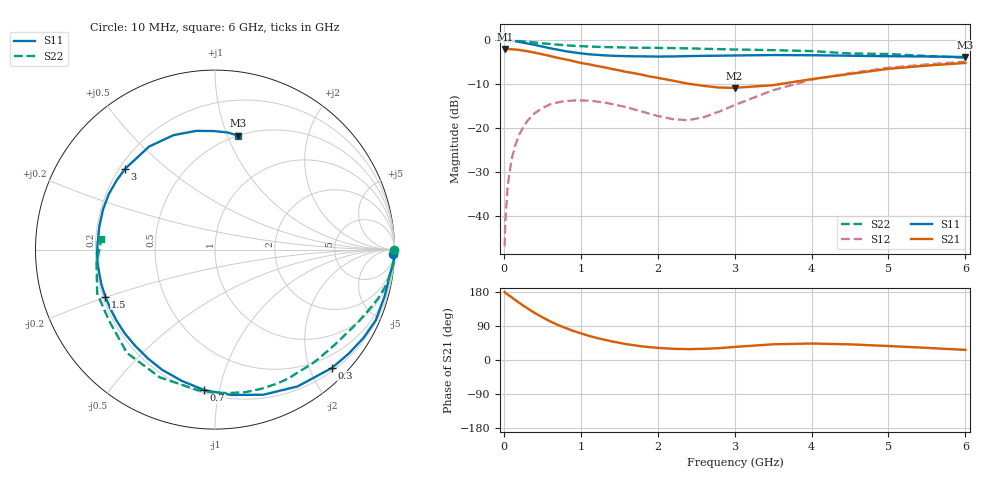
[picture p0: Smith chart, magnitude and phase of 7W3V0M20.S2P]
! Infineon Technologies  Discrete & RF Semiconductors
! BFS17W
! Si NPN RF Bipolar Junction Transistor in SOT323
! VCE = 3 V  IC = 0.2 mA
! Common Emitter S-Parameters:  August  1999
# GHz  S  MA  R  50
!  f  S11  S21  S12  S22
! GHz  MAG  ANG  MAG  ANG  MAG  ANG  MAG  ANG
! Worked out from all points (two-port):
!   36 points, 10 MHz to 6 GHz, reference 50 ohm
!   highest |S21| = -1.93 dB at 20 MHz (marker M1); lowest = -10.8 dB at 3 GHz (marker M2)
!   |S21| within 3 dB of the highest: start of sweep to 952.7 MHz
!   lowest |S11| = -3.8 dB at 6 GHz (marker M3), VSWR 4.68, Z = 25 + j54.7 ohm
!   |S11| at or under -10 dB: nowhere
!   |S22| runs from -3.9 to 0.0 dB; largest |S21 - S12| = 0.8
!   S11 on the Smith chart (normalised r, x): 10 MHz: 26, -66; 300 MHz: 0.25, -2.37; 700 MHz: 0.22, -0.90; 1.5 GHz: 0.21, -0.20; 3 GHz: 0.22, +0.37; 6 GHz: 0.50, +1.09
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0.01  0.9896 -1.5  0.796 179.4  0.0045 88.5  0.9999 0.0
0.02  0.9988 -3.2  0.801 177.2  0.0088 88.9  0.992 -0.8
0.05  0.985 -7.8  0.8 172.7  0.022 85.6  0.9979 -2.3
0.1  0.9804 -15.2  0.793 165.7  0.0438 80.8  0.9975 -4.6
0.2  0.9625 -30.7  0.78 150.8  0.0843 70.9  0.983 -8.9
0.3  0.927 -45.3  0.755 137.2  0.1192 61.6  0.967 -13.0
0.4  0.8904 -58.9  0.726 124.2  0.1479 53.2  0.9481 -16.8
0.5  0.8522 -71.6  0.696 112.9  0.1692 46.0  0.9279 -20.1
0.7  0.785 -94.4  0.634 92.7  0.1965 34.3  0.8962 -26.3
0.9  0.732 -113.6  0.582 77.0  0.2062 24.9  0.8694 -32.2
1.1  0.6963 -129.9  0.536 64.1  0.2057 18.0  0.8535 -37.8
1.5  0.665 -156.8  0.456 45.3  0.1807 10.6  0.8351 -49.4
1.8  0.6585 -173.3  0.405 35.8  0.1544 10.9  0.8256 -58.7
2.2  0.6573 168.6  0.347 29.5  0.1264 24.4  0.8178 -71.3
2.6  0.6677 152.4  0.303 29.4  0.1333 47.8  0.8031 -84.4
3  0.6737 138.1  0.288 34.5  0.1832 61.6  0.7887 -97.1
3.5  0.6814 122.6  0.309 41.4  0.2706 63.5  0.7752 -113.4
4  0.6783 109.9  0.362 43.5  0.3568 57.8  0.7562 -130.5
4.5  0.6698 99.0  0.415 41.3  0.4238 50.4  0.7108 -146.2
5  0.6606 90.8  0.475 36.9  0.4884 43.2  0.7004 -159.6
5.5  0.6564 83.8  0.517 32.0  0.5332 36.2  0.6644 -173.4
6  0.6477 78.5  0.554 26.7  0.5736 29.8  0.6357 174.8
